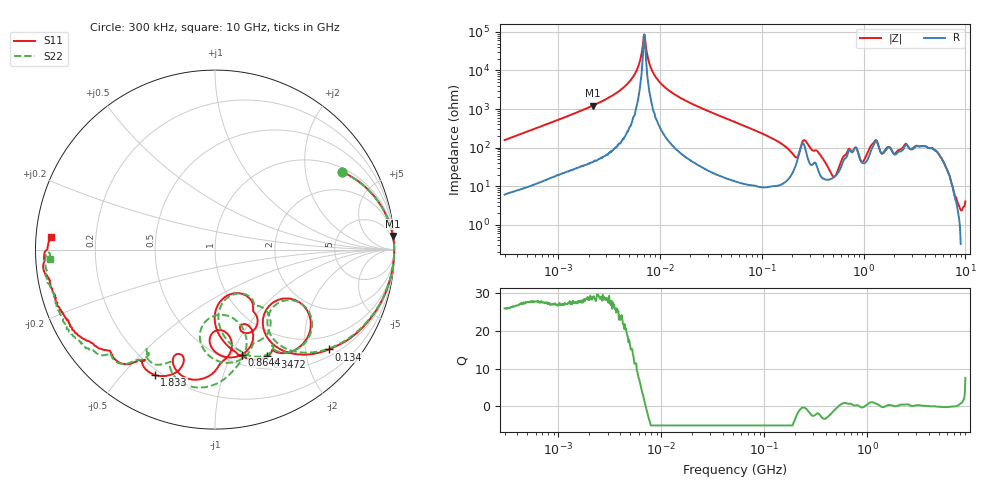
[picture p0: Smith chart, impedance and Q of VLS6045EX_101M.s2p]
! S-Parameter Data Generated by TDK Corporation
! Copyright(C) 2019 TDK Corporation.
! All Rights Reserved.
! TDK P/N: VLS6045EX-101M (Inductor)
! Property: L=100uH at 100kHz
! Size(LxWxT): 6x6x4.5mm
! Model Type: s2p (Touchstone File Format Version 1.0)
! Frequency: DC=Yes Start=0.3MHz Stop=10000MHz 802points Log-sweep
! Model Generated on May 10, 2019
! Port Assignments:
!  1 ---@@@--- 2
! Applicable Conditions:
!  Temperature = 25 degC
!  DC Bias Current = 0 A
!  Small Signal Operation
! Terms and conditions regarding TDK Simulation Models
! (1)This simulation model is being provided solely for informational purposes. Please refer to the specifications of the products in terms of detailed characteristics of such products.
! (2)In no event shall TDK Corporation of any of its subsidiaries be liable for any loss or damage arising, directly or indirectly,
!  From any information contained in this simulation model, including, but not limited to loss or damages arising from any inaccuracies, omissions or errors in connection with such information.
! (3)Any and all copyrights on this simulation model are owned by TDK Corporation.
!  Duplication or redistribution of this simulation model without prior written permission from TDK Corporation is prohibited.
! (4)This simulation model is subject to any modification or change without any prior notice.
! (5)Neither TDK Corporation nor any of its subsidiaries shall make any warranty, express or implied,
!  Including but not limited to the correctness, implied warranties of merchantability and fitness for a particular purpose with respect to this simulation models.
! (6)The use of this simulation model shall be deemed to have consented to the terms and conditions hereof.
# Hz S MA R 50
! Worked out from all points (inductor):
!   801 points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, 300 kHz to 10 GHz, reference 50 ohm
!   read as one part in series: L = 83.2 uH near 318.3 kHz
!   highest Q = 29 at 2.211 MHz (marker M1), where L = 88.7 uH
!   self-resonance near 6.985 MHz
!   S11 on the Smith chart (normalised r, x): 300 kHz: 1.14, +3.16; 134 MHz: 0.65, -2.51; 347.2 MHz: 0.65, -1.39; 864.4 MHz: 0.60, -1.10; 1.833 GHz: 0.18, -0.61; 10 GHz: 0.04, +0.04
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300000  0.8296 31.6  0.5266 -56.2  0.5268 -56.2  0.8294 31.5
1713600  0.9904 6.0  0.1077 -81.9  0.1077 -82.0  0.9904 6.0
2211197  0.9939 4.4  0.08061 -83.6  0.08069 -83.6  0.9939 4.4
5106625  0.9986 0.6  0.01868 -85.6  0.01863 -85.8  0.9987 0.6
6127430  0.9987 -0.1  0.008051 -81.9  0.008116 -81.7  0.9989 -0.1
6985119  0.9988 -0.6  0.00122 -23.0  0.001283 -26.1  0.9989 -0.6
9671944  0.9984 -1.9  0.01817 83.8  0.01819 83.8  0.9985 -1.9
5.477226e7  0.9718 -17.1  0.2088 71.5  0.2088 71.5  0.9721 -16.6
1.340254e8  0.8435 -41.3  0.4864 45.9  0.4864 45.9  0.8469 -40.2
2.351426e8  0.469 -35.5  0.5496 -7.4  0.5497 -7.4  0.4908 -35.0
3.126428e8  0.6584 -59.5  0.5713 11.2  0.5713 11.2  0.6449 -59.4
3.471693e8  0.6628 -63.9  0.5727 8.9  0.5727 8.9  0.649 -61.2
4.687561e8  0.4539 -88.4  0.7631 -12.9  0.7632 -12.9  0.4587 -85.3
5.82867e8  0.2627 -70.9  0.749 -40.3  0.749 -40.3  0.2697 -69.1
7.152593e8  0.4937 -62.9  0.4736 -57.2  0.4736 -57.2  0.5108 -52.5
8.643532e8  0.6041 -75.6  0.4034 -45.9  0.4035 -45.9  0.6351 -83.8
1.038183e9  0.4488 -88.1  0.5843 -69.4  0.5845 -69.4  0.3656 -88.8
1.180962e9  0.6035 -83.5  0.3805 -94.4  0.3806 -94.4  0.5972 -73.7
1.767019e9  0.7549 -111.2  0.2337 -96.0  0.2342 -96.1  0.7044 -114.8
1.832918e9  0.775 -115.7  0.2256 -91.9  0.2261 -92.0  0.7221 -117.6
5.284132e9  0.9244 -159.5  0.05025 -128.8  0.0503 -128.1  0.9319 -153.7
1e10  0.9187 175.6  0.05523 -150.2  0.0551 -150.8  0.9219 -176.7
